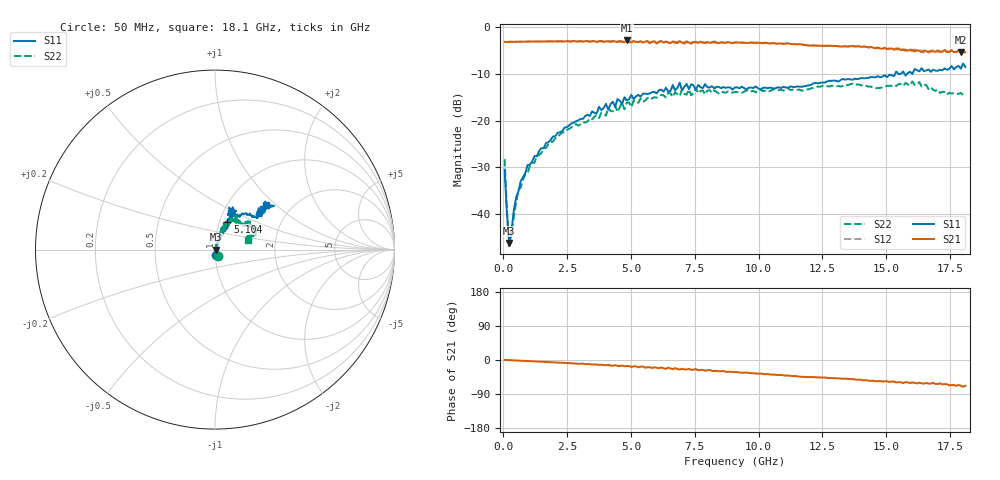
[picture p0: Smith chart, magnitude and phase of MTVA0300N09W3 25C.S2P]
! Network Analyzer HP8720D.06.14 Serial No. US36140669
!  7 Jul 2005  12:33:25
! Frequency  S11  S21  S12  S22
# HZ  S  DB R 50
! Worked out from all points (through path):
!   201 points, 50 MHz to 18.1 GHz, reference 50 ohm
!   highest |S21| = -2.79 dB at 4.833 GHz (marker M1); lowest = -5.3 dB at 17.92 GHz (marker M2)
!   group delay of S21, straight-line fit = 10.7 ps
!   lowest |S11| = -46.3 dB at 230.5 MHz (marker M3), VSWR 1.01, Z = 50.5 - j0.0913 ohm
!   |S11| at or under -10 dB: start of sweep to 15.34 GHz; 15.47962 GHz to 15.51847 GHz (38.85 MHz wide, 0.251 % of centre); 15.72 GHz to 15.81 GHz (92.83 MHz wide, 0.589 % of centre)
!   |S22| runs from -47.0 to -11.6 dB; largest |S21 - S12| = 0.041
!   S11 on the Smith chart (normalised r, x): 50 MHz: 1.01, -0.06; 5.104 GHz: 1.09, +0.35; 18.1 GHz: 1.48, +0.87
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5e7  -30.51 -76.1  -3.09 0.4  -3.07 0.3  -28.29 -62.1
1.4025e8  -39.75 -63.2  -3.13 -0.2  -3.13 -0.2  -39.50 -65.8
2.305e8  -46.30 -10.8  -3.08 -0.4  -3.07 -0.5  -46.97 -27.5
4.11e8  -39.23 57.9  -3.09 -1.1  -3.08 -1.1  -40.64 62.5
5.915e8  -35.18 67.1  -3.06 -1.3  -3.09 -1.5  -35.03 71.6
9.525e8  -29.54 67.2  -3.04 -2.7  -3.01 -2.6  -31.37 73.3
1.58425e9  -25.89 65.5  -3.00 -4.7  -3.00 -4.9  -25.91 73.6
3.1185e9  -19.64 65.4  -3.02 -9.7  -3.04 -10.1  -20.32 72.8
4.83325e9  -15.66 68.8  -2.79 -16.3  -3.07 -17.1  -16.18 61.9
5.104e9  -15.37 66.3  -2.88 -17.0  -3.02 -18.1  -15.70 64.1
6.09675e9  -13.44 63.7  -3.09 -21.6  -2.99 -21.4  -14.91 61.6
6.7285e9  -13.52 70.5  -3.12 -21.3  -3.42 -22.2  -13.87 55.7
6.909e9  -11.84 67.3  -2.95 -25.3  -3.04 -23.2  -14.71 55.6
6.99925e9  -13.53 67.3  -3.23 -23.1  -3.42 -25.4  -13.32 56.1
7.17975e9  -12.12 71.7  -2.98 -25.0  -3.27 -23.4  -14.44 51.4
7.54075e9  -13.39 63.8  -3.20 -24.0  -3.07 -27.3  -13.04 58.4
9.075e9  -12.86 65.2  -3.22 -31.8  -3.18 -32.0  -13.84 46.9
1.21435e10  -11.98 52.5  -3.86 -45.1  -3.81 -45.4  -12.96 42.4
1.512175e10  -10.15 36.9  -4.62 -58.0  -4.40 -57.6  -12.54 34.5
1.6295e10  -9.43 37.1  -5.02 -59.9  -4.96 -63.6  -11.70 25.3
1.79195e10  -8.86 39.1  -5.34 -67.8  -5.17 -68.3  -14.05 21.9
1.81e10  -8.48 41.6  -5.31 -68.2  -5.51 -69.1  -14.26 16.1
